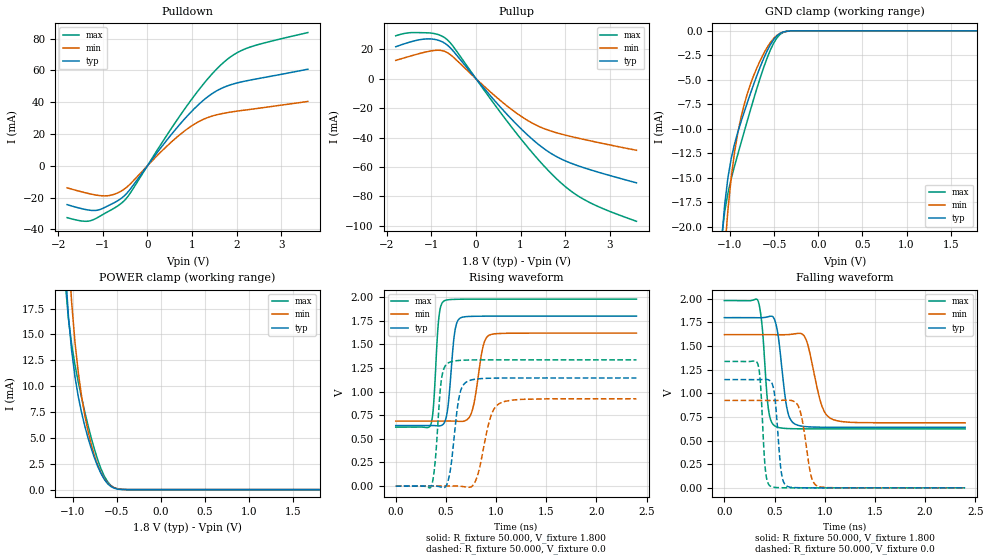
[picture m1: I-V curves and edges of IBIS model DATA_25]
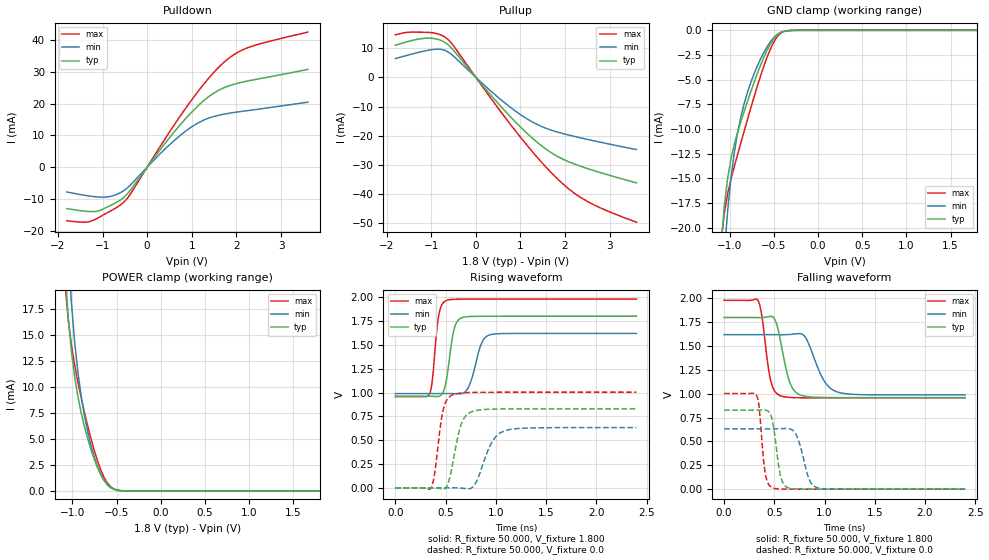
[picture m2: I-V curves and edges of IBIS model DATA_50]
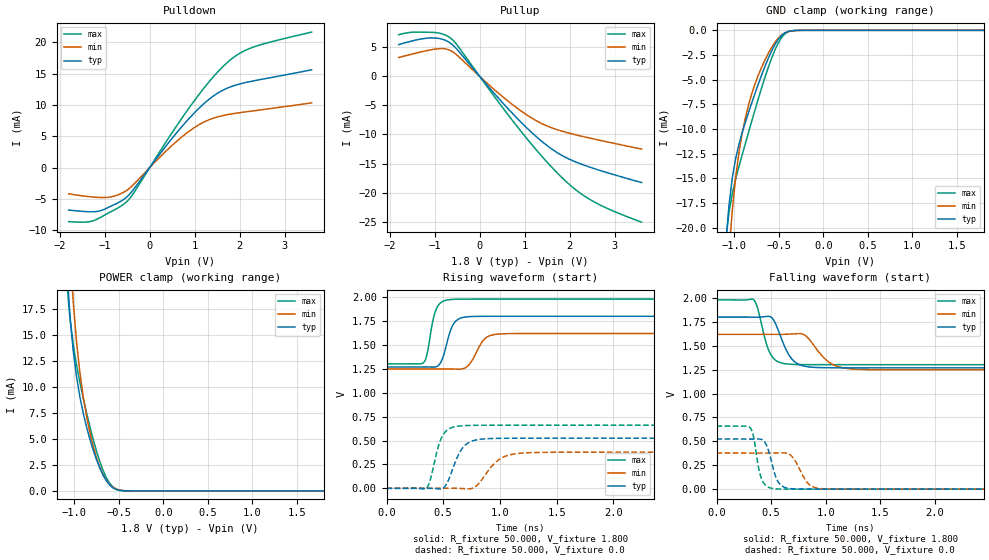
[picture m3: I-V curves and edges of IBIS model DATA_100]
| This Model is valid for Industrial Temperature Range -40C<=Tc<=125C
| Valid for LPSDR-800Mbps operation
| Part Number   VDD/VDDQ   Package   Architecture
| X8: SCB18X128800AF-10E1   1.8 +0.18/-0.18   miniBGA 24L   16M x 8bits
| X16:SCB18X128160AF-10E1   1.8 +0.18/-0.18   miniBGA 24L   8M  x 16bits
| Comment:X8/X16 mode can be configured by Mode Register
[IBIS ver] 5.0
[File name]  usssx128xxae1.ibs
[File Rev]  1.0
[Date]   July 17, 2023
[Source] Simulation of a silicon level SPICE model
[Notes] Revision History:
   Rev 1.0: 08/22/2023
   - First release
[Disclaimer] The IBIS models are for modeling purpose only and are subject
   to change without any notice. UniIC is not responsible for
   any problems the models may cause.
[Copyright] Copyright 2023 UniIC Semiconductors Corp. All rights reserved
|   Component Uniic_128M_LPSDR
[Component] Uniic_128M_LPSDR
[Manufacturer] UniIC Semiconductors Corp
[Package]
| variable   typ   min   max
R_pkg   0.5767   0.3531   0.7590
L_pkg   3.2983nH   2.0138nH   4.7047nH
C_pkg   0.9552pF   0.7789pF   1.2427pF
[Pin]  signal_name   model_name   R_pin   L_pin   C_pin
A2   DQ10   DQ   0.5339   3.0670nH   0.9739pF
A3   CE_N   CE_N   0.3749   2.1956nH   0.7789pF
A4   DQ11   DQ   0.5455   3.1041nH   0.9721pF
A5   DQ12   DQ   0.4956   3.0079nH   0.8178pF
B1   DQ9   DQ   0.6019   3.5461nH   0.9364pF
B2   CLK   CLK   0.3530   2.0138nH   0.8533pF
B3   DQS1   DQ   0.7526   3.7181nH   1.2427pF
B4   DQ13   DQ   0.4982   2.9019nH   0.8357pF
B5   DQ14   DQ   0.5354   3.1357nH   0.7864pF
C1   VSS   Gnd   NA   NA   NA
C2   DQ8   DQ   0.6453   3.6845nH   1.0409pF
C3   DQS0   DQ   0.5006   2.6361nH   1.0173pF
C4   DQ2   DQ   0.7589   4.7046nH   1.1224pF
C5   DQ15   DQ   0.5850   3.0705nH   0.9034pF
D1   VDD   Power   NA   NA   NA
D2   DQ1   DQ   0.5493   3.0081nH   0.9868pF
D3   DQ0   DQ   0.6058   3.5484nH   0.9301pF
D4   DQ3   DQ   0.6182   3.9764nH   0.9922pF
D5   DQ4   DQ   0.6012   3.6086nH   0.8670pF
E1   DQ7   DQ   0.5840   3.3663nH   0.8827pF
E2   DQ6   DQ   0.6809   3.7995nH   1.0960pF
E3   DQ5   DQ   0.7137   3.8728nH   1.0675pF
E4   VDD   Power   NA   NA   NA
E5   VSS   Gnd   NA   NA   NA
|IN   dq_in   dummy
|EN   dq_en   dummy
[Model Selector] DQ
DATA_25   RON=25ohms
DATA_50   RON=50ohms
DATA_100   RON=100ohms
DATA_200   RON=200ohms
DATA_240   RON=240ohms
| Models and submodels in the file (7): DATA_25 (I/O), DATA_50 (I/O), DATA_100 (I/O), DATA_200 (I/O), DATA_240 (I/O), CE_N (Input), CLK (Input)
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|   Model DATA_25
[Model] DATA_25
Model_type I/O
Polarity   Inverting
Enable   Active-High
Vinl =  0.0V
Vinh =  1.800V
Vmeas =  0.900V
Vref =  0.900V
C_comp   1.060pF   1.050pF   1.070pF
[Model Spec]
Vinh   1.800V   1.400V   2.100V
Vinl   0.0V   -0.300V   0.400V
Vmeas   0.900V   0.810V   0.990V
Vref   0.900V   0.810V   0.990V
[Temperature Range]   25.000   0.125k   -40.000
[Voltage Range]   1.800V   1.620V   1.980V
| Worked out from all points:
|   slope of the pulldown table from 0 to 0.27 V, typ, clamps not added: 26.6 ohm
|   slope of the pullup table from 0 to 0.27 V, typ, clamps not added: 27.7 ohm
|   GND clamp passes 1 mA (typ) near -0.51 V on its own axis
|   POWER clamp passes 1 mA (typ) near -0.64 V on its own axis
|   rising waveform, R_fixture 50.000, V_fixture 1.800: 20-80 % time 56.5ps typ, 81.8ps min, 43.7ps max; typ from 0.64 V to 1.8 V
|   rising waveform, R_fixture 50.000, V_fixture 0.0: 20-80 % time 74.6ps typ, 114ps min, 54.6ps max; typ from 0 V to 1.15 V
|   falling waveform, R_fixture 50.000, V_fixture 1.800: 20-80 % time 77ps typ, 120ps min, 55.6ps max; typ from 1.8 V to 0.64 V
|   falling waveform, R_fixture 50.000, V_fixture 0.0: 20-80 % time 52.4ps typ, 80.8ps min, 40.7ps max; typ from 1.15 V to 0 V
[Pulldown]
|Voltage   I(typ)   I(min)   I(max)
-1.8V     -24.38mA   -13.83mA   -32.56mA
-1.415V   -27.29mA   -16.76mA   -34.84mA
-1.14V    -27.99mA   -18.41mA   -32.88mA
-810mV    -24.12mA   -18.4mA    -27.66mA
-535mV    -19.3mA    -14.97mA   -22.35mA
-370mV    -14.14mA   -10.99mA   -16.56mA
400mV     14.86mA    11.37mA    17.65mA
895mV     31.34mA    23.21mA    38.04mA
1.39V     44.18mA    30.73mA    55.85mA
1.83V     50.61mA    33.64mA    67.78mA
2.325V    54.03mA    35.56mA    74.89mA
3.6V      60.78mA    40.51mA    83.81mA
[Pullup]
|Voltage   I(typ)   I(min)   I(max)
-1.8V     21.71mA    12.43mA    29.15mA
-1.515V   24.58mA    14.98mA    31.15mA
-1.13V    26.98mA    18.11mA    31.2mA
-910mV    26.61mA    19.25mA    30.49mA
-690mV    23.89mA    18.44mA    27.6mA
-525mV    19.28mA    15.08mA    22.45mA
300mV     -10.79mA   -8.364mA   -12.7mA
850mV     -29.13mA   -22.06mA   -34.89mA
1.345V    -43.24mA   -31.47mA   -53.17mA
1.785V    -52.58mA   -36.54mA   -67.34mA
2.445V    -60.73mA   -41.43mA   -82.42mA
3.6V      -70.74mA   -48.62mA   -96.87mA
[GND_clamp]
|Voltage   I(typ)   I(min)   I(max)
-1.8V     -271.7mA   -304.3mA   -257.9mA
-1.097V   -21.71mA   -28.04mA   -21.32mA
-1.06V    -17.73mA   -22.52mA   -18.46mA
-1.023V   -14.97mA   -18.24mA   -16.55mA
-986mV    -13.03mA   -14.97mA   -15.09mA
-912mV    -10.37mA   -10.44mA   -12.62mA
-801mV    -7.262mA   -6.333mA   -9.099mA
-690mV    -4.437mA   -3.666mA   -5.721mA
-579mV    -2.043mA   -1.694mA   -2.765mA
-431mV    -248.4uA   -247.4uA   -345.1uA
-283mV    -5.293uA   -10.2uA    -5.65uA
1.8V      0A         0A         0A
[POWER_clamp]
|Voltage   I(typ)   I(min)   I(max)
-1.8V     340.2mA    394mA      317.1mA
-1.086V   21.52mA    29.62mA    20.16mA
-1.049V   16.79mA    23.07mA    16.54mA
-1.012V   13.42mA    18.08mA    14.02mA
-975mV    10.94mA    14.29mA    12.08mA
-938mV    9.034mA    11.39mA    10.43mA
-901mV    7.488mA    9.092mA    8.933mA
-827mV    5.01mA     5.66mA     6.217mA
-716mV    2.228mA    2.327mA    2.865mA
-568mV    301.3uA    355.6uA    397.2uA
-420mV    7.103uA    18.41uA    6.039uA
1.8V      0A         0A         0A
[Ramp]
| variable   typ   min   max
dV/dt_r   0.687/74.860p   0.555/0.114n   0.802/54.976p
dV/dt_f   0.696/77.315p   0.559/0.119n   0.814/55.910p
R_load = 50.000
[Rising Waveform]
R_fixture= 50.000
V_fixture= 1.800
V_fixture_min= 1.620
V_fixture_max= 1.980
|time   V(typ)   V(min)   V(max)
0s        640.4mV    687.8mV    624mV
350ps     641.1mV    688mV      651.2mV
375ps     640.7mV    688mV      830.6mV
431ps     637.1mV    688mV      1.794V
485ps     671.4mV    688.2mV    1.963V
590ps     1.643V     687.6mV    1.978V
648ps     1.783V     684.4mV    1.979V
757ps     1.797V     781.3mV    1.98V
932ps     1.8V       1.598V     1.98V
2.4ns     1.8V       1.62V      1.98V
[Rising Waveform]
R_fixture= 50.000
V_fixture= 0.0
V_fixture_min= 0.0
V_fixture_max= 0.0
|time   V(typ)   V(min)   V(max)
0s        7.256nV    52nV       11.02nV
355ps     645.5uV    103.1uV    -2.392mV
394ps     -153uV     78.95uV    267.3mV
454ps     -11.75mV   56.47uV    1.117V
529ps     85.15mV    340.4uV    1.307V
627ps     916.3mV    -835.5uV   1.33V
719ps     1.111V     -12.52mV   1.335V
805ps     1.133V     79.87mV    1.336V
1.037ns   1.144V     875.9mV    1.337V
2.4ns     1.145V     924.3mV    1.337V
[Falling Waveform]
R_fixture= 50.000
V_fixture= 1.800
V_fixture_min= 1.620
V_fixture_max= 1.980
|time   V(typ)   V(min)   V(max)
0s        1.8V       1.62V      1.98V
338ps     1.799V     1.62V      1.972V
377ps     1.799V     1.62V      1.704V
438ps     1.81V      1.62V      840.6mV
506ps     1.762V     1.62V      652.3mV
620ps     862.1mV    1.62V      627.8mV
708ps     672.1mV    1.63V      625mV
816ps     647mV      1.563V     624.2mV
1.054ns   640.7mV    737.3mV    624mV
2.4ns     640.4mV    687.8mV    624mV
[Falling Waveform]
R_fixture= 50.000
V_fixture= 0.0
V_fixture_min= 0.0
V_fixture_max= 0.0
|time   V(typ)   V(min)   V(max)
0s        1.145V     924.3mV    1.337V
333ps     1.144V     924.2mV    1.311V
409ps     1.147V     924.2mV    190.2mV
457ps     1.132V     924.1mV    18.66mV
501ps     978.6mV    923.9mV    4.994mV
568ps     162.1mV    925.6mV    1.383mV
625ps     16.83mV    927.7mV    548.4uV
747ps     1.53mV     839.3mV    82.75uV
922ps     146uV      21.39mV    5.71uV
2.4ns     7.22nV     53.22nV    11.02nV
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|   Model DATA_50
[Model] DATA_50
Model_type I/O
Polarity   Inverting
Enable   Active-High
Vinl =  0.0V
Vinh =  1.800V
Vmeas =  0.900V
Vref =  0.900V
C_comp   1.060pF   1.050pF   1.070pF
[Model Spec]
Vinh   1.800V   1.400V   2.100V
Vinl   0.0V   -0.300V   0.400V
Vmeas   0.900V   0.810V   0.990V
Vref   0.900V   0.810V   0.990V
[Temperature Range]   25.000   0.125k   -40.000
[Voltage Range]   1.800V   1.620V   1.980V
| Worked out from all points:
|   slope of the pulldown table from 0 to 0.27 V, typ, clamps not added: 52.7 ohm
|   slope of the pullup table from 0 to 0.27 V, typ, clamps not added: 55.1 ohm
|   GND clamp passes 1 mA (typ) near -0.51 V on its own axis
|   POWER clamp passes 1 mA (typ) near -0.64 V on its own axis
|   rising waveform, R_fixture 50.000, V_fixture 1.800: 20-80 % time 70.4ps typ, 98.4ps min, 55.3ps max; typ from 0.959 V to 1.8 V
|   rising waveform, R_fixture 50.000, V_fixture 0.0: 20-80 % time 100ps typ, 146ps min, 74.6ps max; typ from 0 V to 0.829 V
|   falling waveform, R_fixture 50.000, V_fixture 1.800: 20-80 % time 105ps typ, 155ps min, 77.5ps max; typ from 1.8 V to 0.959 V
|   falling waveform, R_fixture 50.000, V_fixture 0.0: 20-80 % time 65.4ps typ, 96ps min, 50.5ps max; typ from 0.829 V to 0 V
[Pulldown]
|Voltage   I(typ)   I(min)   I(max)
-1.8V     -13.05mA   -7.82mA    -16.88mA
-1.36V    -13.94mA   -8.961mA   -17.34mA
-1.085V   -13.77mA   -9.423mA   -15.9mA
-755mV    -11.62mA   -8.966mA   -13.32mA
-480mV    -8.958mA   -6.949mA   -10.41mA
400mV     7.505mA    5.738mA    8.917mA
895mV     15.83mA    11.72mA    19.23mA
1.39V     22.36mA    15.53mA    28.27mA
1.83V     25.66mA    17.01mA    34.38mA
2.05V     26.56mA    17.48mA    36.4mA
2.325V    27.4mA     17.99mA    38.06mA
3.6V      30.87mA    20.52mA    42.64mA
[Pullup]
|Voltage   I(typ)   I(min)   I(max)
-1.8V     10.96mA    6.423mA    14.53mA
-1.515V   12.26mA    7.612mA    15.41mA
-1.075V   13.39mA    9.232mA    15.38mA
-855mV    13.01mA    9.634mA    14.89mA
-635mV    11.33mA    8.805mA    13.12mA
355mV     -6.404mA   -4.955mA   -7.547mA
905mV     -15.55mA   -11.74mA   -18.66mA
1.345V    -21.86mA   -15.92mA   -26.85mA
1.84V     -27.16mA   -18.79mA   -34.92mA
2.17V     -29.45mA   -20.1mA    -39.25mA
2.5V      -31.24mA   -21.25mA   -42.48mA
3.6V      -36.14mA   -24.76mA   -49.6mA
[GND_clamp]
|Voltage   I(typ)   I(min)   I(max)
-1.8V     -271.7mA   -304.3mA   -257.9mA
-1.097V   -21.71mA   -28.04mA   -21.32mA
-1.06V    -17.73mA   -22.52mA   -18.46mA
-1.023V   -14.97mA   -18.24mA   -16.55mA
-986mV    -13.03mA   -14.97mA   -15.09mA
-912mV    -10.37mA   -10.44mA   -12.62mA
-801mV    -7.262mA   -6.333mA   -9.099mA
-690mV    -4.437mA   -3.666mA   -5.721mA
-579mV    -2.043mA   -1.694mA   -2.765mA
-431mV    -248.4uA   -247.4uA   -345.1uA
-283mV    -5.293uA   -10.2uA    -5.65uA
1.8V      0A         0A         0A
[POWER_clamp]
|Voltage   I(typ)   I(min)   I(max)
-1.8V     340.2mA    394mA      317.1mA
-1.086V   21.52mA    29.62mA    20.16mA
-1.049V   16.79mA    23.07mA    16.54mA
-1.012V   13.42mA    18.08mA    14.02mA
-975mV    10.94mA    14.29mA    12.08mA
-938mV    9.034mA    11.39mA    10.43mA
-901mV    7.488mA    9.092mA    8.933mA
-827mV    5.01mA     5.66mA     6.217mA
-716mV    2.228mA    2.327mA    2.865mA
-568mV    301.3uA    355.6uA    397.2uA
-420mV    7.103uA    18.41uA    6.039uA
1.8V      0A         0A         0A
[Ramp]
| variable   typ   min   max
dV/dt_r   0.497/0.100n   0.379/0.145n   0.602/74.943p
dV/dt_f   0.504/0.105n   0.379/0.156n   0.614/77.555p
R_load = 50.000
[Rising Waveform]
R_fixture= 50.000
V_fixture= 1.800
V_fixture_min= 1.620
V_fixture_max= 1.980
|time   V(typ)   V(min)   V(max)
0s        959.5mV    988.2mV    957.4mV
336ps     960.1mV    988.5mV    979.8mV
367ps     959.8mV    988.5mV    1.128V
431ps     959.9mV    988.4mV    1.81V
507ps     1.13V      988.6mV    1.965V
583ps     1.66V      987.8mV    1.977V
669ps     1.787V     991mV      1.979V
862ps     1.799V     1.528V     1.98V
932ps     1.8V       1.602V     1.98V
2.4ns     1.8V       1.62V      1.98V
[Rising Waveform]
R_fixture= 50.000
V_fixture= 0.0
V_fixture_min= 0.0
V_fixture_max= 0.0
|time   V(typ)   V(min)   V(max)
0s        10.43nV    71.14nV    16.62nV
352ps     619.3uV    79.19uV    -6.618mV
387ps     340.4uV    65.08uV    129mV
471ps     -11.83mV   66.49uV    798.5mV
575ps     283.2mV    496.3uV    977.8mV
661ps     683.4mV    -3.469mV   995.4mV
777ps     804.7mV    17.3mV     1.001V
966ps     825.7mV    488.1mV    1.003V
1.103ns   828mV      602.9mV    1.003V
2.4ns     828.7mV    631.9mV    1.003V
[Falling Waveform]
R_fixture= 50.000
V_fixture= 1.800
V_fixture_min= 1.620
V_fixture_max= 1.980
|time   V(typ)   V(min)   V(max)
0s        1.8V       1.62V      1.98V
335ps     1.799V     1.62V      1.984V
378ps     1.799V     1.62V      1.804V
466ps     1.812V     1.62V      1.13V
556ps     1.584V     1.619V     981.7mV
656ps     1.116V     1.622V     962mV
773ps     982mV      1.627V     958.2mV
989ps     961mV      1.148V     957.5mV
1.115ns   959.9mV    1.024V     957.4mV
2.4ns     959.5mV    988.2mV    957.4mV
[Falling Waveform]
R_fixture= 50.000
V_fixture= 0.0
V_fixture_min= 0.0
V_fixture_max= 0.0
|time   V(typ)   V(min)   V(max)
0s        828.7mV    631.9mV    1.003V
325ps     828.3mV    631.8mV    980.4mV
352ps     829.2mV    631.8mV    828.1mV
406ps     830.5mV    631.8mV    191.2mV
480ps     723.7mV    631.6mV    14.48mV
558ps     158.1mV    633.1mV    1.807mV
640ps     13.74mV    634.7mV    405.8uV
717ps     2.321mV    573.2mV    124.3uV
926ps     115.5uV    15.83mV    5.745uV
2.4ns     38.57nV    106.4nV    42.27nV
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|   Model DATA_100
[Model] DATA_100
Model_type I/O
Polarity   Inverting
Enable   Active-High
Vinl =  0.0V
Vinh =  1.800V
Vmeas =  0.900V
Vref =  0.900V
C_comp   1.060pF   1.050pF   1.070pF
[Model Spec]
Vinh   1.800V   1.400V   2.100V
Vinl   0.0V   -0.300V   0.400V
Vmeas   0.900V   0.810V   0.990V
Vref   0.900V   0.810V   0.990V
[Temperature Range]   25.000   0.125k   -40.000
[Voltage Range]   1.800V   1.620V   1.980V
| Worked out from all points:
|   slope of the pulldown table from 0 to 0.27 V, typ, clamps not added: 104 ohm
|   slope of the pullup table from 0 to 0.27 V, typ, clamps not added: 110 ohm
|   GND clamp passes 1 mA (typ) near -0.51 V on its own axis
|   POWER clamp passes 1 mA (typ) near -0.64 V on its own axis
|   rising waveform, R_fixture 50.000, V_fixture 1.800: 20-80 % time 80.1ps typ, 106ps min, 65.7ps max; typ from 1.27 V to 1.8 V
|   rising waveform, R_fixture 50.000, V_fixture 0.0: 20-80 % time 116ps typ, 164ps min, 89.2ps max; typ from 0 V to 0.524 V
|   falling waveform, R_fixture 50.000, V_fixture 1.800: 20-80 % time 126ps typ, 173ps min, 96.1ps max; typ from 1.8 V to 1.27 V
|   falling waveform, R_fixture 50.000, V_fixture 0.0: 20-80 % time 80.4ps typ, 109ps min, 62.6ps max; typ from 0.524 V to 0 V
[Pulldown]
|Voltage   I(typ)   I(min)   I(max)
-1.8V     -6.777mA   -4.19mA    -8.634mA
-1.36V    -7.047mA   -4.628mA   -8.668mA
-1.085V   -6.879mA   -4.78mA    -7.93mA
-755mV    -5.804mA   -4.481mA   -6.65mA
-480mV    -4.501mA   -3.487mA   -5.235mA
-315mV    -3.072mA   -2.383mA   -3.611mA
400mV     3.788mA    2.89mA     4.508mA
895mV     7.995mA    5.904mA    9.722mA
1.39V     11.3mA     7.838mA    14.3mA
1.83V     12.99mA    8.59mA     17.42mA
2.325V    13.88mA    9.087mA    19.31mA
3.6V      15.63mA    10.34mA    21.66mA
[Pullup]
|Voltage   I(typ)   I(min)   I(max)
-1.8V     5.449mA    3.231mA    7.165mA
-1.075V   6.6mA      4.569mA    7.566mA
-855mV    6.43mA     4.765mA    7.342mA
-635mV    5.628mA    4.377mA    6.508mA
-470mV    4.345mA    3.403mA    5.065mA
410mV     -3.678mA   -2.842mA   -4.338mA
905mV     -7.776mA   -5.875mA   -9.321mA
1.345V    -10.95mA   -7.985mA   -13.43mA
1.84V     -13.65mA   -9.452mA   -17.5mA
2.17V     -14.83mA   -10.12mA   -19.72mA
2.5V      -15.75mA   -10.71mA   -21.4mA
3.6V      -18.27mA   -12.5mA    -25.09mA
[GND_clamp]
|Voltage   I(typ)   I(min)   I(max)
-1.8V     -271.7mA   -304.3mA   -257.9mA
-1.097V   -21.71mA   -28.04mA   -21.32mA
-1.06V    -17.73mA   -22.52mA   -18.46mA
-1.023V   -14.97mA   -18.24mA   -16.55mA
-986mV    -13.03mA   -14.97mA   -15.09mA
-912mV    -10.37mA   -10.44mA   -12.62mA
-801mV    -7.262mA   -6.333mA   -9.099mA
-690mV    -4.437mA   -3.666mA   -5.721mA
-579mV    -2.043mA   -1.694mA   -2.765mA
-431mV    -248.4uA   -247.4uA   -345.1uA
-283mV    -5.293uA   -10.2uA    -5.65uA
1.8V      0A         0A         0A
[POWER_clamp]
|Voltage   I(typ)   I(min)   I(max)
-1.8V     340.2mA    394mA      317.1mA
-1.086V   21.52mA    29.62mA    20.16mA
-1.049V   16.79mA    23.07mA    16.54mA
-1.012V   13.42mA    18.08mA    14.02mA
-975mV    10.94mA    14.29mA    12.08mA
-938mV    9.034mA    11.39mA    10.43mA
-901mV    7.488mA    9.092mA    8.933mA
-827mV    5.01mA     5.66mA     6.217mA
-716mV    2.228mA    2.327mA    2.865mA
-568mV    301.3uA    355.6uA    397.2uA
-420mV    7.103uA    18.41uA    6.039uA
1.8V      0A         0A         0A
[Ramp]
| variable   typ   min   max
dV/dt_r   0.315/0.117n   0.227/0.163n   0.396/89.417p
dV/dt_f   0.318/0.127n   0.223/0.174n   0.407/96.192p
R_load = 50.000
[Rising Waveform]
R_fixture= 50.000
V_fixture= 1.800
V_fixture_min= 1.620
V_fixture_max= 1.980
|time   V(typ)   V(min)   V(max)
0s        1.269V     1.249V     1.302V
327ps     1.27V      1.249V     1.316V
356ps     1.27V      1.249V     1.397V
439ps     1.272V     1.249V     1.876V
492ps     1.353V     1.249V     1.953V
586ps     1.711V     1.248V     1.977V
721ps     1.795V     1.286V     1.98V
885ps     1.8V       1.582V     1.98V
1.074ns   1.8V       1.619V     1.98V
10ns      1.8V       1.62V      1.98V
[Rising Waveform]
R_fixture= 50.000
V_fixture= 0.0
V_fixture_min= 0.0
V_fixture_max= 0.0
|time   V(typ)   V(min)   V(max)
0s        13.61nV    88.88nV    22.46nV
351ps     584uV      52.35uV    -1.723mV
382ps     583.3uV    45.31uV    75.31mV
451ps     -5.181mV   10.28uV    414.3mV
496ps     -1.065mV   155.5uV    554.8mV
685ps     442.2mV    -3.683mV   655.6mV
788ps     505.7mV    21.51mV    659mV
1.018ns   523.2mV    319.4mV    660.1mV
1.268ns   524.3mV    373.5mV    660.1mV
10ns      524.3mV    377.9mV    660.1mV
[Falling Waveform]
R_fixture= 50.000
V_fixture= 1.800
V_fixture_min= 1.620
V_fixture_max= 1.980
|time   V(typ)   V(min)   V(max)
0s        1.8V       1.62V      1.98V
344ps     1.799V     1.62V      1.978V
377ps     1.799V     1.62V      1.892V
493ps     1.805V     1.62V      1.417V
563ps     1.672V     1.619V     1.334V
681ps     1.375V     1.623V     1.307V
813ps     1.285V     1.609V     1.303V
1.065ns   1.27V      1.305V     1.302V
1.305ns   1.269V     1.253V     1.302V
10ns      1.269V     1.249V     1.302V
[Falling Waveform]
R_fixture= 50.000
V_fixture= 0.0
V_fixture_min= 0.0
V_fixture_max= 0.0
|time   V(typ)   V(min)   V(max)
0s        524.3mV    377.9mV    660.1mV
308ps     524mV      377.9mV    643.7mV
333ps     524mV      377.9mV    579.9mV
420ps     516.1mV    377.8mV    88.65mV
464ps     444.5mV    377.8mV    27.11mV
556ps     95.54mV    378.6mV    2.583mV
676ps     5.803mV    358.2mV    196.6uV
837ps     284.4uV    62.53mV    12.17uV
987ps     31.62uV    3.694mV    1.179uV
10ns      17.84nV    92.98nV    26.48nV
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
